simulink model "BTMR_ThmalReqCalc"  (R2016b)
settings: Solver=FixedStepDiscrete  StartTime=0.0  StopTime=10.0  FixedStep=0.1  RelTol=1e-3  EnableMultiTasking=on
undefined symbols (not defined in the file or in its folder): BMS_cntThmStbNum_C, BTMR_cntThmalReqVal_C, BTMR_flgCoolPwrCal_C, BTMR_pChrgClntPwrLv1_C, BTMR_pChrgClntPwrLv2_C, BTMR_pChrgClntPwrLv3_C, BTMR_pChrgClntPwrLv4_C, BTMR_pChrgClntPwrLv5_C, BTMR_pChrgClntPwrLv6_C, BTMR_pCoolPwrVal_C, BTMR_pHtgACPwrReq_C, BTMR_pHtgDCPwrReq_C, BTMR_pHtgDrvPwrReq_C, BTMR_pHtgsStage1_CUR, BTMR_pHtgsStage2_CUR, BTMR_pNormClntPwrLv1_C, BTMR_pNormClntPwrLv2_C, BTMR_pNormClntPwrLv3_C, BTMR_r861BrsDrvSoc_C, BTMR_r861HtgDrvSoc_C, BTMR_r891BrsDrvSoc_C, BTMR_r891HtgDrvSoc_C, BTMR_rCoolClbFlg_C, BTMR_rFlashClbFlg_C, BTMR_rHeatClbFlg_C, BTMR_t861BrsDiffLv0Temp_C, BTMR_t861BrsDiffLv1Temp_C, BTMR_t861CoolChrgAces2Temp_C, BTMR_t861CoolChrgAces3Temp_C, BTMR_t861CoolChrgAcesTemp_C, BTMR_t861CoolChrgDiffDebTemp_C, BTMR_t861CoolChrgEndDiffTemp_C, BTMR_t861CoolChrgExitLv2Temp_C, BTMR_t861CoolChrgExitLv3Temp_C, BTMR_t861CoolChrgExitTemp_C, BTMR_t861CoolChrgIntLv0Temp_C, BTMR_t861CoolChrgIntLv1Temp_C, BTMR_t861CoolChrgIntLv2Temp_C, BTMR_t861CoolChrgIntLv3Temp_C, BTMR_t861CoolChrgIntLv4Temp_C, BTMR_t861CoolChrgIntLv5Temp_C, BTMR_t861CoolDCDebTemp_C, BTMR_t861CoolNormAcesTemp_C, BTMR_t861CoolNormDiffDebTemp_C, BTMR_t861CoolNormEndDiffTemp_C, BTMR_t861CoolNormExitLv2Temp_C, BTMR_t861CoolNormExitLv3Temp_C, BTMR_t861CoolNormExitTemp_C, BTMR_t861CoolNormIntLv0Temp_C, BTMR_t861CoolNormIntLv1Temp_C, BTMR_t861CoolNormLv2Temp_C, BTMR_t861CoolNormLv3Temp_C, BTMR_t861HtgACDiffDebTemp_C, BTMR_t861HtgACEndDiffTemp_C, BTMR_t861HtgACStartHiTemp_C, BTMR_t861HtgACStartLoTemp_C, BTMR_t861HtgACStopTemp_C, BTMR_t861HtgDCDiffDebTemp_C, BTMR_t861HtgDCEndDiffTemp_C, BTMR_t861HtgDCIntLv0Temp_C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
libraries: AIWAYS_Powertrain_BMS_lib x78, simulink x9
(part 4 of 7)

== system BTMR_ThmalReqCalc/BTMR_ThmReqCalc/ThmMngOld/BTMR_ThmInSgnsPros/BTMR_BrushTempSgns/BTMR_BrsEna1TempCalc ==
  BSPR_tCellTempMin : Inport
  BSPR_tCellTempMax : Inport  Port=2
  BMSDebounceStartZero : AIWAYS_Powertrain_BMS_lib/Debounce & Delay/BMSDebounceStartZero
  Constant13 : Constant  Value=BTMR_t861CoolChrgAcesTemp_C
  Constant17 : Constant  Value=BTMR_t861HtgDCStartHiTemp_C
  Constant29 : Constant  Value=BTMR_tiTempBase_C
  Constant30 : Constant  Value=BTMR_tiTempDebs_C
  Logical Operator2 : Logic  AllPortsSameDT=off  OutDataTypeStr=boolean
  Relational Operator8 : RelationalOperator  OutDataTypeStr=boolean  RndMeth=Simplest
  Relational Operator9 : RelationalOperator  Operator=<  OutDataTypeStr=boolean  RndMeth=Simplest
  BTMR_flgBrsEna1Temp : Outport
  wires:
  Relational Operator8/1 -> Logical Operator2/1
  Relational Operator9/1 -> Logical Operator2/2
  Constant13/1 -> Relational Operator9/2
  Constant17/1 -> Relational Operator8/2
  BSPR_tCellTempMin/1 -> Relational Operator8/1
  BSPR_tCellTempMax/1 -> Relational Operator9/1
  Logical Operator2/1 -> BMSDebounceStartZero/1
  BMSDebounceStartZero/1 -> BTMR_flgBrsEna1Temp/1
  Constant29/1 -> BMSDebounceStartZero/5, BMSDebounceStartZero/3
  Constant30/1 -> BMSDebounceStartZero/4, BMSDebounceStartZero/2

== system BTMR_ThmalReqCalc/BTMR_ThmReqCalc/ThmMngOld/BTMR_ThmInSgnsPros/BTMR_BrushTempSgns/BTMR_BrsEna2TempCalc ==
  BSPR_tCellTempMin : Inport
  BSPR_tCellTempMax : Inport  Port=2
  BMSDebounceStartZero : AIWAYS_Powertrain_BMS_lib/Debounce & Delay/BMSDebounceStartZero
  Constant14 : Constant  Value=BTMR_t861HtgACStartHiTemp_C
  Constant16 : Constant  Value=BTMR_t861CoolNormAcesTemp_C
  Constant29 : Constant  Value=BTMR_tiTempBase_C
  Constant30 : Constant  Value=BTMR_tiTempDebs_C
  Logical Operator3 : Logic  AllPortsSameDT=off  OutDataTypeStr=boolean
  Relational Operator10 : RelationalOperator  OutDataTypeStr=boolean  RndMeth=Simplest
  Relational Operator11 : RelationalOperator  Operator=<  OutDataTypeStr=boolean  RndMeth=Simplest
  BTMR_flgBrsEna2Temp : Outport
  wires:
  BMSDebounceStartZero/1 -> BTMR_flgBrsEna2Temp/1
  BSPR_tCellTempMax/1 -> Relational Operator11/1
  BSPR_tCellTempMin/1 -> Relational Operator10/1
  Logical Operator3/1 -> BMSDebounceStartZero/1
  Relational Operator10/1 -> Logical Operator3/1
  Relational Operator11/1 -> Logical Operator3/2
  Constant14/1 -> Relational Operator10/2
  Constant16/1 -> Relational Operator11/2
  Constant29/1 -> BMSDebounceStartZero/5, BMSDebounceStartZero/3
  Constant30/1 -> BMSDebounceStartZero/4, BMSDebounceStartZero/2

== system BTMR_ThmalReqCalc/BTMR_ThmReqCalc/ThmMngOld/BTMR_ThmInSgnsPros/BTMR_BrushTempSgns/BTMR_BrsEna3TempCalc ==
  BSPR_tCellTempMin : Inport
  BSPR_tCellTempMax : Inport  Port=2
  BMSDebounceStartZero : AIWAYS_Powertrain_BMS_lib/Debounce & Delay/BMSDebounceStartZero
  Constant19 : Constant  Value=BTMR_t861CoolNormAcesTemp_C
  Constant20 : Constant  Value=BTMR_t861HtgDrvStartHiTemp_C
  Constant29 : Constant  Value=BTMR_tiTempBase_C
  Constant30 : Constant  Value=BTMR_tiTempDebs_C
  Logical Operator4 : Logic  AllPortsSameDT=off  OutDataTypeStr=boolean
  Relational Operator12 : RelationalOperator  Operator=>  OutDataTypeStr=boolean  RndMeth=Simplest
  Relational Operator13 : RelationalOperator  Operator=<  OutDataTypeStr=boolean  RndMeth=Simplest
  BTMR_flgBrsEna3Temp : Outport
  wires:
  BSPR_tCellTempMax/1 -> Relational Operator13/1
  BMSDebounceStartZero/1 -> BTMR_flgBrsEna3Temp/1
  Relational Operator12/1 -> Logical Operator4/1
  Constant19/1 -> Relational Operator13/2
  Relational Operator13/1 -> Logical Operator4/2
  Constant20/1 -> Relational Operator12/2
  Logical Operator4/1 -> BMSDebounceStartZero/1
  BSPR_tCellTempMin/1 -> Relational Operator12/1
  Constant29/1 -> BMSDebounceStartZero/5, BMSDebounceStartZero/3
  Constant30/1 -> BMSDebounceStartZero/4, BMSDebounceStartZero/2

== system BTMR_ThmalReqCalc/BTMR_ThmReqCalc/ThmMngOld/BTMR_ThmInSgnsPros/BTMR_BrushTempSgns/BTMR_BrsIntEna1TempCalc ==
  BSPR_tClntUsT : Inport
  BMSDebounceStartZero : AIWAYS_Powertrain_BMS_lib/Debounce & Delay/BMSDebounceStartZero
  Constant13 : Constant  Value=BTMR_t861CoolChrgAcesTemp_C
  Constant17 : Constant  Value=BTMR_t861HtgDCStartHiTemp_C
  Constant29 : Constant  Value=BTMR_tiTempBase_C
  Constant30 : Constant  Value=BTMR_tiTempDebs_C
  Logical Operator2 : Logic  AllPortsSameDT=off  OutDataTypeStr=boolean
  Relational Operator8 : RelationalOperator  OutDataTypeStr=boolean  RndMeth=Simplest
  Relational Operator9 : RelationalOperator  Operator=<  OutDataTypeStr=boolean  RndMeth=Simplest
  BTMR_flgBrsIntEna1Temp : Outport
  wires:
  BMSDebounceStartZero/1 -> BTMR_flgBrsIntEna1Temp/1
  Logical Operator2/1 -> BMSDebounceStartZero/1
  BSPR_tClntUsT/1 -> Relational Operator9/1, Relational Operator8/1
  Constant17/1 -> Relational Operator8/2
  Constant13/1 -> Relational Operator9/2
  Relational Operator9/1 -> Logical Operator2/2
  Relational Operator8/1 -> Logical Operator2/1
  Constant29/1 -> BMSDebounceStartZero/5, BMSDebounceStartZero/3
  Constant30/1 -> BMSDebounceStartZero/4, BMSDebounceStartZero/2

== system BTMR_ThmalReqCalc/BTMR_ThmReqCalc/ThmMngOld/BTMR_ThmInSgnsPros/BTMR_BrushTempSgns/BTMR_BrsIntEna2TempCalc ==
  BSPR_tClntUsT : Inport
  BMSDebounceStartZero : AIWAYS_Powertrain_BMS_lib/Debounce & Delay/BMSDebounceStartZero
  Constant14 : Constant  Value=BTMR_t861HtgACStartHiTemp_C
  Constant16 : Constant  Value=BTMR_t861CoolNormAcesTemp_C
  Constant29 : Constant  Value=BTMR_tiTempBase_C
  Constant30 : Constant  Value=BTMR_tiTempDebs_C
  Logical Operator3 : Logic  AllPortsSameDT=off  OutDataTypeStr=boolean
  Relational Operator10 : RelationalOperator  OutDataTypeStr=boolean  RndMeth=Simplest
  Relational Operator11 : RelationalOperator  Operator=<  OutDataTypeStr=boolean  RndMeth=Simplest
  BTMR_flgBrsIntEna2Temp : Outport
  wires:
  Constant16/1 -> Relational Operator11/2
  Constant14/1 -> Relational Operator10/2
  Relational Operator11/1 -> Logical Operator3/2
  Relational Operator10/1 -> Logical Operator3/1
  Logical Operator3/1 -> BMSDebounceStartZero/1
  BSPR_tClntUsT/1 -> Relational Operator11/1, Relational Operator10/1
  BMSDebounceStartZero/1 -> BTMR_flgBrsIntEna2Temp/1
  Constant29/1 -> BMSDebounceStartZero/5, BMSDebounceStartZero/3
  Constant30/1 -> BMSDebounceStartZero/4, BMSDebounceStartZero/2

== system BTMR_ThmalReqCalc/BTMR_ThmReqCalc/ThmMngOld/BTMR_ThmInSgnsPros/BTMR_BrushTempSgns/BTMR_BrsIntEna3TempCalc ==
  BSPR_tClntUsT : Inport
  BMSDebounceStartZero : AIWAYS_Powertrain_BMS_lib/Debounce & Delay/BMSDebounceStartZero
  Constant19 : Constant  Value=BTMR_t861CoolNormAcesTemp_C
  Constant20 : Constant  Value=BTMR_t861HtgDrvStartHiTemp_C
  Constant29 : Constant  Value=BTMR_tiTempBase_C
  Constant30 : Constant  Value=BTMR_tiTempDebs_C
  Logical Operator4 : Logic  AllPortsSameDT=off  OutDataTypeStr=boolean
  Relational Operator12 : RelationalOperator  Operator=>  OutDataTypeStr=boolean  RndMeth=Simplest
  Relational Operator13 : RelationalOperator  Operator=<  OutDataTypeStr=boolean  RndMeth=Simplest
  BTMR_flgBrsIntEna3Temp : Outport
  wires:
  Logical Operator4/1 -> BMSDebounceStartZero/1
  Constant20/1 -> Relational Operator12/2
  Relational Operator13/1 -> Logical Operator4/2
  Constant19/1 -> Relational Operator13/2
  Relational Operator12/1 -> Logical Operator4/1
  BMSDebounceStartZero/1 -> BTMR_flgBrsIntEna3Temp/1
  BSPR_tClntUsT/1 -> Relational Operator13/1, Relational Operator12/1
  Constant29/1 -> BMSDebounceStartZero/5, BMSDebounceStartZero/3
  Constant30/1 -> BMSDebounceStartZero/4, BMSDebounceStartZero/2

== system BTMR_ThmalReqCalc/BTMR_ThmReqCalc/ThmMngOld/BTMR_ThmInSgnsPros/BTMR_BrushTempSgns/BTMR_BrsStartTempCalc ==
  BSPR_tCellTempMin : Inport
  BSPR_tCellTempMax : Inport  Port=2
  BSPR_tClntUsT : Inport  Port=3
  Add : Sum  Inputs=+-
  Add1 : Sum  Inputs=+-
  Add2 : Sum  Inputs=+-
  BMSDebounceStartZero : AIWAYS_Powertrain_BMS_lib/Debounce & Delay/BMSDebounceStartZero
  Constant1 : Constant  Value=BTMR_tBrsCellClntDvtTemp_C
  Constant2 : Constant  Value=BTMR_t861BrsDiffLv1Temp_C
  Constant29 : Constant  Value=BTMR_tiTempBase_C
  Constant3 : Constant  Value=BTMR_tBrsMinCellTempThre_C
  Constant30 : Constant  Value=BTMR_tiTempDebs_C
  Constant4 : Constant  Value=BTMR_tBrsCellClntDvtTemp_C
  Logical Operator4 : Logic  Inputs=4  AllPortsSameDT=off  OutDataTypeStr=boolean
  Relational Operator1 : RelationalOperator  Operator=<  OutDataTypeStr=boolean  RndMeth=Simplest
  Relational Operator2 : RelationalOperator  OutDataTypeStr=boolean  RndMeth=Simplest
  Relational Operator3 : RelationalOperator  Operator=<  OutDataTypeStr=boolean  RndMeth=Simplest
  Relational Operator4 : RelationalOperator  OutDataTypeStr=boolean  RndMeth=Simplest
  BTMR_flgBrsStartTemp : Outport
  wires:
  BMSDebounceStartZero/1 -> BTMR_flgBrsStartTemp/1
  Add/1 -> Relational Operator2/1
  Constant2/1 -> Relational Operator2/2
  Relational Operator2/1 -> Logical Operator4/1
  BSPR_tCellTempMax/1 -> Add2/2, Add/1
  BSPR_tCellTempMin/1 -> Relational Operator4/1, Add/2, Add1/1
  Constant29/1 -> BMSDebounceStartZero/5, BMSDebounceStartZero/3
  Constant30/1 -> BMSDebounceStartZero/4, BMSDebounceStartZero/2
  Relational Operator1/1 -> Logical Operator4/2
  Constant1/1 -> Relational Operator1/2
  Relational Operator3/1 -> Logical Operator4/3
  Add1/1 -> Relational Operator1/1
  Constant4/1 -> Relational Operator3/2
  Add2/1 -> Relational Operator3/1
  BSPR_tClntUsT/1 -> Add2/1, Add1/2
  Logical Operator4/1 -> BMSDebounceStartZero/1
  Constant3/1 -> Relational Operator4/2
  Relational Operator4/1 -> Logical Operator4/4

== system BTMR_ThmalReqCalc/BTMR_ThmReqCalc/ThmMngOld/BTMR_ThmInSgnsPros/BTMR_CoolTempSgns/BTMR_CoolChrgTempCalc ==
  BSPR_tCellTempMax : Inport
  BSPR_tClntUsT : Inport  Port=2
  BTMR_CoolChrgInTempCalc : Subsystem
  BTMR_CoolChrgIntTempCalc : Subsystem
  Bus Creator : BusCreator  Inputs=2
  BTMR_flgCoolChrgTempSgns : Outport
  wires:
  BSPR_tClntUsT/1 -> BTMR_CoolChrgIntTempCalc/1(BSPR_tClntUsT)
  BSPR_tCellTempMax/1 -> BTMR_CoolChrgInTempCalc/1(BSPR_tCellTempMax)
  BTMR_CoolChrgInTempCalc/1(BTMR_flgCoolChrgInTempSgns) -> Bus Creator/1
  BTMR_CoolChrgIntTempCalc/1(BTMR_flgCoolChrgIntTempSgns) -> Bus Creator/2
  Bus Creator/1 -> BTMR_flgCoolChrgTempSgns/1  "BTMR_flgCoolChrgTempSgns"

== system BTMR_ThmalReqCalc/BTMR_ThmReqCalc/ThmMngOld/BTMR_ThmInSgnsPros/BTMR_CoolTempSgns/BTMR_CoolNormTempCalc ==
  BSPR_tCellTempMax : Inport
  BSPR_tClntUsT : Inport  Port=2
  BTMR_CoolNormInTempCalc : Subsystem
  BTMR_CoolNormIntTempCalc : Subsystem
  Bus Creator2 : BusCreator  Inputs=2
  BTMR_flgCoolNormTempSgns : Outport
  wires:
  Bus Creator2/1 -> BTMR_flgCoolNormTempSgns/1  "BTMR_flgCoolNormTempSgns"
  BSPR_tCellTempMax/1 -> BTMR_CoolNormInTempCalc/1(BSPR_tCellTempMax)
  BTMR_CoolNormInTempCalc/1(BTMR_flgCoolNormInTempSgns) -> Bus Creator2/1
  BSPR_tClntUsT/1 -> BTMR_CoolNormIntTempCalc/1(BSPR_tClntUsT)
  BTMR_CoolNormIntTempCalc/1(BTMR_flgCoolNormIntTempSgns) -> Bus Creator2/2

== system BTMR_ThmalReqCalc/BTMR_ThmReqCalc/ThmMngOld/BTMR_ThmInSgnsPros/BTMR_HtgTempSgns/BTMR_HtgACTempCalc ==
  BSPR_tCellTempMin : Inport
  BTMR_HtgACDnaTempCalc : Subsystem
  Bus Creator : BusCreator  Inputs=1
  BTMR_flgHtgACTempSgns : Outport
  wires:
  BTMR_HtgACDnaTempCalc/1(BTMR_flgHtgACDnaTemp) -> Bus Creator/1  "BTMR_flgHtgACDnaTemp"
  BSPR_tCellTempMin/1 -> BTMR_HtgACDnaTempCalc/1(BSPR_tCellTempMin)
  Bus Creator/1 -> BTMR_flgHtgACTempSgns/1  "BTMR_flgHtgACTempSgns"

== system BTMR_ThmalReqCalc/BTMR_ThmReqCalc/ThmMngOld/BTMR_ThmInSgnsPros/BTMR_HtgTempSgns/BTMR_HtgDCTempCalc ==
  BSPR_tCellTempMin : Inport
  BSPR_tCellTempMax : Inport  Port=2
  BSPR_tClntUsT : Inport  Port=3
  BTMR_HtgDCDnaTempCalc : Subsystem
  BTMR_HtgDCStage2EnaTempCalc : Subsystem
  BTMR_HtgDCStage2PowRedTempCalc : Subsystem
  BTMR_HtgDCStage2PowResTempCalc : Subsystem
  BTMR_HtgDCStage3EnaTempCalc : Subsystem
  BTMR_HtgDCStage3PowRedTempCalc : Subsystem
  BTMR_HtgDCStage3PowResTempCalc : Subsystem
  Bus Creator : BusCreator  Inputs=2
  Bus Creator1 : BusCreator  Inputs=5
  Bus Creator2 : BusCreator  Inputs=2
  BTMR_flgHtgDCTempSgns : Outport
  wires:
  BSPR_tClntUsT/1 -> BTMR_HtgDCStage2PowRedTempCalc/1(BSPR_tClntUsT), BTMR_HtgDCStage3PowResTempCalc/1(BSPR_tClntUsT), BTMR_HtgDCStage3PowRedTempCalc/1(BSPR_tClntUsT), BTMR_HtgDCStage2PowResTempCalc/1(BSPR_tClntUsT), BTMR_HtgDCStage2EnaTempCalc/1(BSPR_tClntUsT)
  BSPR_tCellTempMax/1 -> BTMR_HtgDCDnaTempCalc/2(BSPR_tCellTempMax), BTMR_HtgDCStage3EnaTempCalc/2(BSPR_tCellTempMax)
  BTMR_HtgDCDnaTempCalc/1(BTMR_flgHtgDCDnaTemp) -> Bus Creator/2  "BTMR_flgHtgDCDnaTemp"
  BTMR_HtgDCStage3EnaTempCalc/1(BTMR_flgHtgDCStage3EnaTemp) -> Bus Creator/1  "BTMR_flgHtgDCStage3EnaTemp"
  BTMR_HtgDCStage2EnaTempCalc/1(BTMR_flgHtgDCStage2EnaTemp) -> Bus Creator1/1  "BTMR_flgHtgDCStage2EnaTemp"
  BSPR_tCellTempMin/1 -> BTMR_HtgDCDnaTempCalc/1(BSPR_tCellTempMin), BTMR_HtgDCStage3EnaTempCalc/1(BSPR_tCellTempMin)
  BTMR_HtgDCStage2PowRedTempCalc/1(BTMR_flgHtgDCStage2PowRedTemp) -> Bus Creator1/2  "BTMR_HtgDCStage2PowRedTemp"
  BTMR_HtgDCStage2PowResTempCalc/1(BTMR_flgHtgDCStage2PowResTemp) -> Bus Creator1/3  "BTMR_HtgDCStage2PowResTemp"
  BTMR_HtgDCStage3PowRedTempCalc/1(BTMR_flgHtgDCStage3PowRedTemp) -> Bus Creator1/4  "BTMR_HtgDCStage3PowRedTemp"
  BTMR_HtgDCStage3PowResTempCalc/1(BTMR_flgHtgDCStage3PowResTemp) -> Bus Creator1/5  "BTMR_HtgDCStage3PowResTemp"
  Bus Creator/1 -> Bus Creator2/1  "BTMR_flgHtgDCInTempSgns"
  Bus Creator1/1 -> Bus Creator2/2  "BTMR_flgHtgDCIntTempSgns"
  Bus Creator2/1 -> BTMR_flgHtgDCTempSgns/1  "BTMR_flgHtgDCTempSgns"

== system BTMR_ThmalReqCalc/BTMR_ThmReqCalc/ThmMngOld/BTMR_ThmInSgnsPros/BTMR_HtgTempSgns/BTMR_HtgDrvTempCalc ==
  BSPR_tCellTempMin : Inport
  BTMR_HtgDrvDnaTempCalc : Subsystem
  Bus Creator : BusCreator  Inputs=1
  BTMR_flgHtgDrvTempSgns : Outport
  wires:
  BTMR_HtgDrvDnaTempCalc/1(BTMR_flgHtgDrvDnaTemp) -> Bus Creator/1  "BTMR_flgHtgDrvDnaTemp"
  BSPR_tCellTempMin/1 -> BTMR_HtgDrvDnaTempCalc/1(BSPR_tCellTempMin)
  Bus Creator/1 -> BTMR_flgHtgDrvTempSgns/1  "BTMR_flgHtgDrvTempSgns"

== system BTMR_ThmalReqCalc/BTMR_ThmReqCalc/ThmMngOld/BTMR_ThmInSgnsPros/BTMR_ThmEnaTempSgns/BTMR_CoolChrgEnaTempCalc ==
  BSPR_tCellTempMin : Inport
  BSPR_tCellTempMax : Inport  Port=2
  Add : Sum
  Add1 : Sum  Inputs=+-
  Add2 : Sum  Inputs=+-
  BMSDebounceStartZero : AIWAYS_Powertrain_BMS_lib/Debounce & Delay/BMSDebounceStartZero
  Constant1 : Constant  Value=BTMR_t861HtgDCStopTemp_C
  Constant2 : Constant  Value=BTMR_t861CoolDCDebTemp_C
  Constant27 : Constant  Value=BTMR_t861CoolChrgAcesTemp_C
  Constant29 : Constant  Value=BTMR_tiTempBase_C
  Constant3 : Constant  Value=BTMR_t861CoolChrgDiffDebTemp_C
  Constant30 : Constant  Value=BTMR_tiTempDebs_C
  Constant4 : Constant  Value=BTMR_t861CoolChrgEndDiffTemp_C
  Logical Operator : Logic  Inputs=3  AllPortsSameDT=off  OutDataTypeStr=boolean
  Relational Operator1 : RelationalOperator  OutDataTypeStr=boolean  RndMeth=Simplest
  Relational Operator19 : RelationalOperator  OutDataTypeStr=boolean  RndMeth=Simplest
  Relational Operator2 : RelationalOperator  Operator=<  OutDataTypeStr=boolean  RndMeth=Simplest
  BTMR_flgCoolChrgEnaTemp : Outport
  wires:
  Logical Operator/1 -> BMSDebounceStartZero/1
  BSPR_tCellTempMax/1 -> Relational Operator19/1, Add1/1
  Constant27/1 -> Relational Operator19/2
  BMSDebounceStartZero/1 -> BTMR_flgCoolChrgEnaTemp/1
  Constant29/1 -> BMSDebounceStartZero/5, BMSDebounceStartZero/3
  Constant30/1 -> BMSDebounceStartZero/4, BMSDebounceStartZero/2
  BSPR_tCellTempMin/1 -> Relational Operator1/1, Add1/2
  Add/1 -> Relational Operator1/2
  Constant2/1 -> Add/2
  Constant1/1 -> Add/1
  Relational Operator19/1 -> Logical Operator/1
  Relational Operator1/1 -> Logical Operator/3
  Constant4/1 -> Add2/1
  Add2/1 -> Relational Operator2/2
  Constant3/1 -> Add2/2
  Add1/1 -> Relational Operator2/1
  Relational Operator2/1 -> Logical Operator/2

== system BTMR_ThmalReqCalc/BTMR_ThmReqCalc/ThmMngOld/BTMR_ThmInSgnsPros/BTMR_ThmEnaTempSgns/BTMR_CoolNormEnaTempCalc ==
  BSPR_tCellTempMin : Inport
  BSPR_tCellTempMax : Inport  Port=2
  Add1 : Sum  Inputs=+-
  Add2 : Sum  Inputs=+-
  BMSDebounceStartZero : AIWAYS_Powertrain_BMS_lib/Debounce & Delay/BMSDebounceStartZero
  Constant28 : Constant  Value=BTMR_t861CoolNormAcesTemp_C
  Constant29 : Constant  Value=BTMR_tiTempBase_C
  Constant3 : Constant  Value=BTMR_t861CoolNormDiffDebTemp_C
  Constant30 : Constant  Value=BTMR_tiTempDebs_C
  Constant4 : Constant  Value=BTMR_t861CoolNormEndDiffTemp_C
  Logical Operator : Logic  AllPortsSameDT=off  OutDataTypeStr=boolean
  Relational Operator2 : RelationalOperator  Operator=<  OutDataTypeStr=boolean  RndMeth=Simplest
  Relational Operator20 : RelationalOperator  OutDataTypeStr=boolean  RndMeth=Simplest
  BTMR_flgCoolNormEnaTemp : Outport
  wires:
  BMSDebounceStartZero/1 -> BTMR_flgCoolNormEnaTemp/1  "BTMR_flgCoolNormEnaTemp"
  Constant28/1 -> Relational Operator20/2
  BSPR_tCellTempMax/1 -> Add1/1, Relational Operator20/1
  Constant29/1 -> BMSDebounceStartZero/5, BMSDebounceStartZero/3
  Constant30/1 -> BMSDebounceStartZero/4, BMSDebounceStartZero/2
  Add2/1 -> Relational Operator2/2
  BSPR_tCellTempMin/1 -> Add1/2
  Constant3/1 -> Add2/2
  Add1/1 -> Relational Operator2/1
  Constant4/1 -> Add2/1
  Relational Operator20/1 -> Logical Operator/1
  Relational Operator2/1 -> Logical Operator/2  "BTMR_flgTempDiff"
  Logical Operator/1 -> BMSDebounceStartZero/1

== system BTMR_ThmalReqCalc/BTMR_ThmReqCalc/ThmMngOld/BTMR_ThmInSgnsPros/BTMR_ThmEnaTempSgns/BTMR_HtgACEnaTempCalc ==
  BSPR_tCellTempMin : Inport
  BSPR_tCellTempMax : Inport  Port=2
  BMSDebounceStartZero : AIWAYS_Powertrain_BMS_lib/Debounce & Delay/BMSDebounceStartZero
  Constant1 : Constant  Value=BTMR_t861HtgACDiffDebTemp_C
  Constant2 : Constant  Value=BTMR_t861HtgACEndDiffTemp_C
  Constant23 : Constant  Value=BTMR_t861HtgACStartLoTemp_C
  Constant24 : Constant  Value=BTMR_t861HtgACStartHiTemp_C
  Constant29 : Constant  Value=BTMR_tiTempBase_C
  Constant30 : Constant  Value=BTMR_tiTempDebs_C
  Logical Operator6 : Logic  Inputs=3  AllPortsSameDT=off  OutDataTypeStr=boolean
  Relational Operator1 : RelationalOperator  Operator=<  OutDataTypeStr=boolean  RndMeth=Simplest
  Relational Operator14 : RelationalOperator  OutDataTypeStr=boolean  RndMeth=Simplest
  Relational Operator15 : RelationalOperator  Operator=<  OutDataTypeStr=boolean  RndMeth=Simplest
  Sum1 : Sum  Inputs=+-  OutDataTypeStr=Inherit: Inherit via back propagation  RndMeth=Zero
  Sum2 : Sum  Inputs=+-  OutDataTypeStr=Inherit: Inherit via back propagation  RndMeth=Zero
  BTMR_flgHtgACEnaTemp : Outport
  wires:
  BMSDebounceStartZero/1 -> BTMR_flgHtgACEnaTemp/1
  Relational Operator14/1 -> Logical Operator6/2
  Constant24/1 -> Relational Operator15/2
  Constant23/1 -> Relational Operator14/2
  Relational Operator15/1 -> Logical Operator6/3
  Logical Operator6/1 -> BMSDebounceStartZero/1
  Constant29/1 -> BMSDebounceStartZero/5, BMSDebounceStartZero/3
  Constant30/1 -> BMSDebounceStartZero/4, BMSDebounceStartZero/2
  Sum2/1 -> Relational Operator1/2
  Constant1/1 -> Sum2/2
  BSPR_tCellTempMax/1 -> Sum1/1
  Sum1/1 -> Relational Operator1/1
  BSPR_tCellTempMin/1 -> Sum1/2, Relational Operator15/1, Relational Operator14/1
  Relational Operator1/1 -> Logical Operator6/1
  Constant2/1 -> Sum2/1

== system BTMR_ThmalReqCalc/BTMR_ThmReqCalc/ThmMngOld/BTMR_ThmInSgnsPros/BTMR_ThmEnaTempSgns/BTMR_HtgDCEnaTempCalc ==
  BSPR_tCellTempMin : Inport
  BSPR_tCellTempMax : Inport  Port=2
  BMSDebounceStartZero : AIWAYS_Powertrain_BMS_lib/Debounce & Delay/BMSDebounceStartZero
  Constant1 : Constant  Value=BTMR_t861HtgDCDiffDebTemp_C
  Constant2 : Constant  Value=BTMR_t861HtgDCEndDiffTemp_C
  Constant23 : Constant  Value=BTMR_t861HtgDCStopTemp2_C
  Constant25 : Constant  Value=BTMR_t861HtgDCStartHiTemp_C
  Constant26 : Constant  Value=BTMR_t861HtgDCStartLoTemp_C
  Constant29 : Constant  Value=BTMR_tiTempBase_C
  Constant30 : Constant  Value=BTMR_tiTempDebs_C
  Constant5 : Constant  Value=BTMR_tHtgDCMaxTempDeb_C
  Logical Operator6 : Logic  Inputs=4  AllPortsSameDT=off  OutDataTypeStr=boolean
  Relational Operator1 : RelationalOperator  Operator=<  OutDataTypeStr=boolean  RndMeth=Simplest
  Relational Operator16 : RelationalOperator  Operator=>  OutDataTypeStr=boolean  RndMeth=Simplest
  Relational Operator17 : RelationalOperator  Operator=<  OutDataTypeStr=boolean  RndMeth=Simplest
  Relational Operator2 : RelationalOperator  Operator=<  OutDataTypeStr=boolean  RndMeth=Simplest
  Sum1 : Sum  Inputs=+-  OutDataTypeStr=Inherit: Inherit via back propagation  RndMeth=Zero
  Sum2 : Sum  Inputs=+-  OutDataTypeStr=Inherit: Inherit via back propagation  RndMeth=Zero
  Sum3 : Sum  Inputs=+-  OutDataTypeStr=Inherit: Inherit via back propagation  RndMeth=Zero
  BTMR_flgHtgDCEnaTemp : Outport
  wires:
  BMSDebounceStartZero/1 -> BTMR_flgHtgDCEnaTemp/1
  BSPR_tCellTempMin/1 -> Sum1/2, Relational Operator17/1, Relational Operator16/1
  Constant25/1 -> Relational Operator17/2
  Relational Operator17/1 -> Logical Operator6/4
  Constant26/1 -> Relational Operator16/2
  Relational Operator16/1 -> Logical Operator6/3
  Logical Operator6/1 -> BMSDebounceStartZero/1
  Constant30/1 -> BMSDebounceStartZero/4, BMSDebounceStartZero/2
  Constant29/1 -> BMSDebounceStartZero/5, BMSDebounceStartZero/3
  Sum1/1 -> Relational Operator1/1
  Constant1/1 -> Sum2/2
  Constant2/1 -> Sum2/1
  Sum2/1 -> Relational Operator1/2
  Relational Operator1/1 -> Logical Operator6/2
  Sum3/1 -> Relational Operator2/2
  Constant5/1 -> Sum3/2
  Constant23/1 -> Sum3/1
  BSPR_tCellTempMax/1 -> Relational Operator2/1, Sum1/1
  Relational Operator2/1 -> Logical Operator6/1

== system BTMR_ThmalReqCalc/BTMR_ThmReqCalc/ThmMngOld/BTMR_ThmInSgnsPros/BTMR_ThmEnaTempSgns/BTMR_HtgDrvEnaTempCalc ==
  BSPR_tCellTempMin : Inport
  BSPR_tCellTempMax : Inport  Port=2
  BMSDebounceStartZero : AIWAYS_Powertrain_BMS_lib/Debounce & Delay/BMSDebounceStartZero
  Constant1 : Constant  Value=BTMR_t861HtgDrvDiffDebTemp_C
  Constant2 : Constant  Value=BTMR_t861HtgDrvEndDiffTemp_C
  Constant21 : Constant  Value=BTMR_t861HtgDrvStartLoTemp_C
  Constant22 : Constant  Value=BTMR_t861HtgDrvStartHiTemp_C
  Constant29 : Constant  Value=BTMR_tiTempBase_C
  Constant30 : Constant  Value=BTMR_tiTempDebs_C
  Logical Operator6 : Logic  Inputs=3  AllPortsSameDT=off  OutDataTypeStr=boolean
  Relational Operator1 : RelationalOperator  OutDataTypeStr=boolean  RndMeth=Simplest
  Relational Operator18 : RelationalOperator  Operator=<=  OutDataTypeStr=boolean  RndMeth=Simplest
  Relational Operator2 : RelationalOperator  Operator=<  OutDataTypeStr=boolean  RndMeth=Simplest
  Sum1 : Sum  Inputs=+-  OutDataTypeStr=Inherit: Inherit via back propagation  RndMeth=Zero
  Sum2 : Sum  Inputs=+-  OutDataTypeStr=Inherit: Inherit via back propagation  RndMeth=Zero
  BTMR_flgHtgDrvEnaTemp : Outport
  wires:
  Constant22/1 -> Relational Operator18/2
  BMSDebounceStartZero/1 -> BTMR_flgHtgDrvEnaTemp/1
  Logical Operator6/1 -> BMSDebounceStartZero/1
  Constant21/1 -> Relational Operator1/2
  Relational Operator18/1 -> Logical Operator6/2
  Relational Operator1/1 -> Logical Operator6/3
  Constant29/1 -> BMSDebounceStartZero/5, BMSDebounceStartZero/3
  Constant30/1 -> BMSDebounceStartZero/4, BMSDebounceStartZero/2
  BSPR_tCellTempMax/1 -> Sum1/1
  Sum1/1 -> Relational Operator2/1
  Constant2/1 -> Sum2/1
  Sum2/1 -> Relational Operator2/2
  Constant1/1 -> Sum2/2
  BSPR_tCellTempMin/1 -> Relational Operator18/1, Sum1/2, Relational Operator1/1
  Relational Operator2/1 -> Logical Operator6/1

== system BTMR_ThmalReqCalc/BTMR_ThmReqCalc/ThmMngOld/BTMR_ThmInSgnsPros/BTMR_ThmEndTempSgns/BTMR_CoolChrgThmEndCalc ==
  BTMR_flgBMSSgns : Inport
  BSPR_tCellTempMax : Inport  Port=2
  BSPR_tCellTempMin : Inport  Port=3
  Add : Sum  Inputs=+-
  BMSDebounceStartZero : AIWAYS_Powertrain_BMS_lib/Debounce & Delay/BMSDebounceStartZero
  Bus Selector : BusSelector  OutputSignals=BTMR_flgBMSDChrg
  Constant14 : Constant  Value=BTMR_t861CoolChrgEndDiffTemp_C
  Constant29 : Constant  Value=BTMR_tiTempBase_C
  Constant30 : Constant  Value=BTMR_tiTempDebs_C
  Logical Operator1 : Logic  AllPortsSameDT=off  OutDataTypeStr=boolean
  Relational Operator3 : RelationalOperator  OutDataTypeStr=boolean  RndMeth=Simplest
  BTMR_CoolChrgThmEnd : Outport
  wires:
  BMSDebounceStartZero/1 -> Logical Operator1/2
  BSPR_tCellTempMin/1 -> Add/2
  Add/1 -> Relational Operator3/1
  Constant14/1 -> Relational Operator3/2
  BSPR_tCellTempMax/1 -> Add/1
  Relational Operator3/1 -> BMSDebounceStartZero/1
  BTMR_flgBMSSgns/1 -> Bus Selector/1
  Bus Selector/1 -> Logical Operator1/1  "<BTMR_flgBMSDChrg>"
  Logical Operator1/1 -> BTMR_CoolChrgThmEnd/1
  Constant29/1 -> BMSDebounceStartZero/5, BMSDebounceStartZero/3
  Constant30/1 -> BMSDebounceStartZero/4, BMSDebounceStartZero/2

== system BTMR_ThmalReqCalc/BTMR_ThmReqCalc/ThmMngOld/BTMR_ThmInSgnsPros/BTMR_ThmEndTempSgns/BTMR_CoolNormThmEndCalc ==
  BTMR_flgBMSSgns : Inport
  BSPR_tCellTempMax : Inport  Port=2
  BSPR_tCellTempMin : Inport  Port=3
  Add : Sum  Inputs=+-
  BMSDebounceStartZero : AIWAYS_Powertrain_BMS_lib/Debounce & Delay/BMSDebounceStartZero
  Bus Selector : BusSelector  OutputSignals=BTMR_flgBMSAChrg,BTMR_flgBMSDrv
  Constant14 : Constant  Value=BTMR_t861CoolNormEndDiffTemp_C
  Constant29 : Constant  Value=BTMR_tiTempBase_C
  Constant30 : Constant  Value=BTMR_tiTempDebs_C
  Logical Operator1 : Logic  AllPortsSameDT=off  OutDataTypeStr=boolean
  Logical Operator2 : Logic  Operator=OR  AllPortsSameDT=off  OutDataTypeStr=boolean
  Relational Operator3 : RelationalOperator  OutDataTypeStr=boolean  RndMeth=Simplest
  BTMR_CoolNormThmEnd : Outport
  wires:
  BTMR_flgBMSSgns/1 -> Bus Selector/1
  Relational Operator3/1 -> BMSDebounceStartZero/1
  BSPR_tCellTempMax/1 -> Add/1
  Constant14/1 -> Relational Operator3/2
  Add/1 -> Relational Operator3/1
  BSPR_tCellTempMin/1 -> Add/2
  BMSDebounceStartZero/1 -> Logical Operator1/2
  Bus Selector/1 -> Logical Operator2/1  "<BTMR_flgBMSAChrg>"
  Bus Selector/2 -> Logical Operator2/2  "<BTMR_flgBMSDrv>"
  Logical Operator2/1 -> Logical Operator1/1
  Logical Operator1/1 -> BTMR_CoolNormThmEnd/1
  Constant29/1 -> BMSDebounceStartZero/5, BMSDebounceStartZero/3
  Constant30/1 -> BMSDebounceStartZero/4, BMSDebounceStartZero/2

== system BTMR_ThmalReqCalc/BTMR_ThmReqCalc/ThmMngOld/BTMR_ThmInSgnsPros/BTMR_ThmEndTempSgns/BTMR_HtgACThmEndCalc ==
  BTMR_flgBMSSgns : Inport
  BSPR_tCellTempMax : Inport  Port=2
  BSPR_tCellTempMin : Inport  Port=3
  BCMR_bAcChrgHeatFbd : Inport  Port=4
  Add : Sum  Inputs=+-
  BMSDebounceStartZero : AIWAYS_Powertrain_BMS_lib/Debounce & Delay/BMSDebounceStartZero
  Bus Selector : BusSelector  OutputSignals=BTMR_flgBMSAChrg
  Constant14 : Constant  Value=BTMR_t861HtgACEndDiffTemp_C
  Constant29 : Constant  Value=BTMR_tiTempBase_C
  Constant30 : Constant  Value=BTMR_tiTempDebs_C
  Logical Operator1 : Logic  AllPortsSameDT=off  OutDataTypeStr=boolean
  Logical Operator3 : Logic  Operator=OR  AllPortsSameDT=off  OutDataTypeStr=boolean
  Relational Operator3 : RelationalOperator  OutDataTypeStr=boolean  RndMeth=Simplest
  BTMR_HtgACThmEnd : Outport
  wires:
  BMSDebounceStartZero/1 -> Logical Operator3/1
  BSPR_tCellTempMin/1 -> Add/2
  Add/1 -> Relational Operator3/1
  Constant14/1 -> Relational Operator3/2
  BSPR_tCellTempMax/1 -> Add/1
  Relational Operator3/1 -> BMSDebounceStartZero/1
  BTMR_flgBMSSgns/1 -> Bus Selector/1
  Bus Selector/1 -> Logical Operator1/1  "<BTMR_flgBMSAChrg>"
  BCMR_bAcChrgHeatFbd/1 -> Logical Operator3/2
  Logical Operator3/1 -> Logical Operator1/2
  Logical Operator1/1 -> BTMR_HtgACThmEnd/1
  Constant29/1 -> BMSDebounceStartZero/3, BMSDebounceStartZero/5
  Constant30/1 -> BMSDebounceStartZero/2, BMSDebounceStartZero/4

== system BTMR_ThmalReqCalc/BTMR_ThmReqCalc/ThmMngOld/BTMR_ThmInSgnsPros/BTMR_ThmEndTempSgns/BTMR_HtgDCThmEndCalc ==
  BTMR_flgBMSSgns : Inport
  BSPR_tCellTempMax : Inport  Port=2
  BSPR_tCellTempMin : Inport  Port=3
  Add : Sum  Inputs=+-
  BMSDebounceStartZero : AIWAYS_Powertrain_BMS_lib/Debounce & Delay/BMSDebounceStartZero
  Bus Selector : BusSelector  OutputSignals=BTMR_flgBMSDChrg
  Constant14 : Constant  Value=BTMR_t861HtgDCEndDiffTemp_C
  Constant29 : Constant  Value=BTMR_tiTempBase_C
  Constant30 : Constant  Value=BTMR_tiTempDebs_C
  Logical Operator1 : Logic  AllPortsSameDT=off  OutDataTypeStr=boolean
  Relational Operator3 : RelationalOperator  OutDataTypeStr=boolean  RndMeth=Simplest
  BTMR_HtgDCThmEnd : Outport
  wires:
  Bus Selector/1 -> Logical Operator1/1  "<BTMR_flgBMSDChrg>"
  BTMR_flgBMSSgns/1 -> Bus Selector/1
  Relational Operator3/1 -> BMSDebounceStartZero/1
  BSPR_tCellTempMax/1 -> Add/1
  Constant14/1 -> Relational Operator3/2
  Add/1 -> Relational Operator3/1
  BSPR_tCellTempMin/1 -> Add/2
  Logical Operator1/1 -> BTMR_HtgDCThmEnd/1
  BMSDebounceStartZero/1 -> Logical Operator1/2
  Constant29/1 -> BMSDebounceStartZero/5, BMSDebounceStartZero/3
  Constant30/1 -> BMSDebounceStartZero/4, BMSDebounceStartZero/2

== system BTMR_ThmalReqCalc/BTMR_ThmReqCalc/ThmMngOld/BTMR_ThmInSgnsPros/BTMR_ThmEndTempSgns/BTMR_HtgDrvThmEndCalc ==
  BTMR_flgBMSSgns : Inport
  BSPR_tCellTempMax : Inport  Port=2
  BSPR_tCellTempMin : Inport  Port=3
  Add : Sum  Inputs=+-
  BMSDebounceStartZero : AIWAYS_Powertrain_BMS_lib/Debounce & Delay/BMSDebounceStartZero
  Bus Selector : BusSelector  OutputSignals=BTMR_flgBMSDrv
  Constant14 : Constant  Value=BTMR_t861HtgDrvEndDiffTemp_C
  Constant29 : Constant  Value=BTMR_tiTempBase_C
  Constant30 : Constant  Value=BTMR_tiTempDebs_C
  Logical Operator1 : Logic  AllPortsSameDT=off  OutDataTypeStr=boolean
  Relational Operator3 : RelationalOperator  OutDataTypeStr=boolean  RndMeth=Simplest
  BTMR_HtgDrvThmEnd : Outport
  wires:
  BMSDebounceStartZero/1 -> Logical Operator1/2
  Logical Operator1/1 -> BTMR_HtgDrvThmEnd/1
  BSPR_tCellTempMin/1 -> Add/2
  Add/1 -> Relational Operator3/1
  Constant14/1 -> Relational Operator3/2
  BSPR_tCellTempMax/1 -> Add/1
  Relational Operator3/1 -> BMSDebounceStartZero/1
  BTMR_flgBMSSgns/1 -> Bus Selector/1
  Bus Selector/1 -> Logical Operator1/1  "<BTMR_flgBMSDrv>"
  Constant29/1 -> BMSDebounceStartZero/5, BMSDebounceStartZero/3
  Constant30/1 -> BMSDebounceStartZero/4, BMSDebounceStartZero/2

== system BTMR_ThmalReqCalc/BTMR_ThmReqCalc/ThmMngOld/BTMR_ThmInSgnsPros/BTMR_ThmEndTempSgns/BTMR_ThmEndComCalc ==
  BMCR_stBmsModeCtrl : Inport
  DSMR_stFaultRank : Inport  Port=2
  COMR_bLeadAcidChgHvOn : Inport  Port=3
  Data Type Conversion2 : DataTypeConversion  OutDataTypeStr=uint8
  Detect Change : simulink/Logic and Bit Operations/Detect Change  vinit=0  OutDataTypeStr=boolean
  Logical Operator10 : Logic  Operator=OR  Inputs=3  AllPortsSameDT=off  OutDataTypeStr=boolean
  Relational Operator2 : RelationalOperator  OutDataTypeStr=boolean  RndMeth=Simplest
  stBms_DChrg2 : Constant  Value=enmBmsFaultLvl.FaultLv3  OutDataTypeStr=Enum: enmBmsFaultLvl
  BTMR_ThmEndCom : Outport
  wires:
  DSMR_stFaultRank/1 -> Relational Operator2/1
  Relational Operator2/1 -> Logical Operator10/2
  Data Type Conversion2/1 -> Relational Operator2/2
  Logical Operator10/1 -> BTMR_ThmEndCom/1
  COMR_bLeadAcidChgHvOn/1 -> Logical Operator10/3
  stBms_DChrg2/1 -> Data Type Conversion2/1
  Detect Change/1 -> Logical Operator10/1
  BMCR_stBmsModeCtrl/1 -> Detect Change/1

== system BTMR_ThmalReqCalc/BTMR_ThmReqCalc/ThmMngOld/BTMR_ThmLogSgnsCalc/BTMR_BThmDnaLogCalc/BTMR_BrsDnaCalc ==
  BTMR_flgBrsLogSgns : Inport
  Bus Selector : BusSelector  OutputSignals=BTMR_flgBrsInTempSgns
  Bus Selector2 : BusSelector  OutputSignals=BTMR_flgBrsDnaTemp
  BTMR_flgBrsDna : Outport
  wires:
  Bus Selector2/1 -> BTMR_flgBrsDna/1  "<BTMR_flgBrsDnaTemp>"
  BTMR_flgBrsLogSgns/1 -> Bus Selector/1
  Bus Selector/1 -> Bus Selector2/1  "<BTMR_flgBrsInTempSgns>"

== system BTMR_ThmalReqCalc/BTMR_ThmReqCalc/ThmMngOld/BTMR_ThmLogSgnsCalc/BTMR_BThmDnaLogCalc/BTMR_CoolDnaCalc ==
  BTMR_flgCoolLogSgns : Inport
  Bus Selector : BusSelector  OutputSignals=BTMR_flgCoolNormTempSgns
  Bus Selector1 : BusSelector  OutputSignals=BTMR_flgCoolNormInTempSgns
  Bus Selector2 : BusSelector  OutputSignals=BTMR_flgCoolChrgTempSgns
  Bus Selector3 : BusSelector  OutputSignals=BTMR_flgCoolChrgInTempSgns
  Bus Selector4 : BusSelector  OutputSignals=BTMR_flgCoolNormDnaTemp
  Bus Selector5 : BusSelector  OutputSignals=BTMR_flgCoolChrgDnaTemp
  BTMR_flgCoolNormDna : Outport
  BTMR_flgCoolChrgDna : Outport  Port=2
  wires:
  Bus Selector3/1 -> Bus Selector5/1  "<BTMR_flgCoolChrgInTempSgns>"
  Bus Selector2/1 -> Bus Selector3/1  "<BTMR_flgCoolChrgTempSgns>"
  Bus Selector/1 -> Bus Selector1/1  "<BTMR_flgCoolNormTempSgns>"
  BTMR_flgCoolLogSgns/1 -> Bus Selector/1, Bus Selector2/1
  Bus Selector1/1 -> Bus Selector4/1  "<BTMR_flgCoolNormInTempSgns>"
  Bus Selector4/1 -> BTMR_flgCoolNormDna/1  "<BTMR_flgCoolNormDnaTemp>"
  Bus Selector5/1 -> BTMR_flgCoolChrgDna/1  "<BTMR_flgCoolChrgDnaTemp>"

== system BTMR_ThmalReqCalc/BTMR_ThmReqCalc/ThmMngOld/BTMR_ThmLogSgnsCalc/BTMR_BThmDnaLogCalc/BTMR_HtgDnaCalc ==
  BTMR_flgHtgLogSgns : Inport
  BTMR_flgSOCSgns : Inport  Port=2
  Bus Selector : BusSelector  OutputSignals=BTMR_flgHtgDCTempSgns
  Bus Selector1 : BusSelector  OutputSignals=BTMR_flgHtgDCInTempSgns.BTMR_flgHtgDCDnaTemp
  Bus Selector2 : BusSelector  OutputSignals=BTMR_flgHtgACTempSgns
  Bus Selector3 : BusSelector  OutputSignals=BTMR_flgHtgACDnaTemp
  Bus Selector4 : BusSelector  OutputSignals=BTMR_flgHtgDrvTempSgns
  Bus Selector5 : BusSelector  OutputSignals=BTMR_flgHtgDrvDnaTemp
  Bus Selector6 : BusSelector  OutputSignals=BTMR_flgHtgDrvSOC
  Logical Operator1 : Logic  Operator=NOT  AllPortsSameDT=off  OutDataTypeStr=boolean
  Logical Operator3 : Logic  Operator=OR  AllPortsSameDT=off  OutDataTypeStr=boolean
  BTMR_flgHtgDCDna : Outport
  BTMR_flgHtgACDna : Outport  Port=2
  BTMR_flgHtgDrvDna : Outport  Port=3
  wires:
  Bus Selector1/1 -> BTMR_flgHtgDCDna/1  "<BTMR_flgHtgDCDnaTemp>"
  Bus Selector4/1 -> Bus Selector5/1  "<BTMR_flgHtgDrvTempSgns>"
  BTMR_flgHtgLogSgns/1 -> Bus Selector2/1, Bus Selector4/1, Bus Selector/1
  Bus Selector5/1 -> Logical Operator3/1  "<BTMR_flgHtgDrvDnaTemp>"
  Bus Selector/1 -> Bus Selector1/1  "<BTMR_flgHtgDCTempSgns>"
  Bus Selector2/1 -> Bus Selector3/1  "<BTMR_flgHtgACTempSgns>"
  Bus Selector3/1 -> BTMR_flgHtgACDna/1  "<BTMR_flgHtgACDnaTemp>"
  BTMR_flgSOCSgns/1 -> Bus Selector6/1
  Bus Selector6/1 -> Logical Operator1/1  "<BTMR_flgHtgDrvSOC>"
  Logical Operator3/1 -> BTMR_flgHtgDrvDna/1
  Logical Operator1/1 -> Logical Operator3/2

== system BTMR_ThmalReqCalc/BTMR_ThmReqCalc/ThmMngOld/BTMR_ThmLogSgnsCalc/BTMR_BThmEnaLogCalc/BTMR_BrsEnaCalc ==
  BTMR_flgBrsLogSgns : Inport
  Bus Selector : BusSelector  OutputSignals=BTMR_flgBrsEnaLogSgns
  Bus Selector1 : BusSelector  OutputSignals=BTMR_flgBrsEna
  BTMR_flgBrsEna : Outport
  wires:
  BTMR_flgBrsLogSgns/1 -> Bus Selector/1
  Bus Selector/1 -> Bus Selector1/1  "<BTMR_flgBrsEnaLogSgns>"
  Bus Selector1/1 -> BTMR_flgBrsEna/1  "<BTMR_flgBrsEna>"

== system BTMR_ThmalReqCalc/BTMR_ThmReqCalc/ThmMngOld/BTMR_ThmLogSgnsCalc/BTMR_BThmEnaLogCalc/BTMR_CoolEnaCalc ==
  BTMR_flgCoolLogSgns : Inport
  Bus Selector : BusSelector  OutputSignals=BTMR_flgCoolNormLogSgns
  Bus Selector1 : BusSelector  OutputSignals=BTMR_flgCoolNormEna
  Bus Selector2 : BusSelector  OutputSignals=BTMR_flgCoolChrgLogSgns
  Bus Selector3 : BusSelector  OutputSignals=BTMR_flgCoolChrgEna
  BTMR_flgCoolNormEna : Outport
  BTMR_flgCoolChrgEna : Outport  Port=2
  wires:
  Bus Selector1/1 -> BTMR_flgCoolNormEna/1  "<BTMR_flgCoolNormEna>"
  BTMR_flgCoolLogSgns/1 -> Bus Selector2/1, Bus Selector/1
  Bus Selector/1 -> Bus Selector1/1  "<BTMR_flgCoolNormLogSgns>"
  Bus Selector2/1 -> Bus Selector3/1  "<BTMR_flgCoolChrgLogSgns>"
  Bus Selector3/1 -> BTMR_flgCoolChrgEna/1  "<BTMR_flgCoolChrgEna>"

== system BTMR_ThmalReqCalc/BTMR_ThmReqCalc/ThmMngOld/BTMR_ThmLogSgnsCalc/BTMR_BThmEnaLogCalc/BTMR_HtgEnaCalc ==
  BTMR_flgHtgLogSgns : Inport
  BTMR_flgSOCSgns : Inport  Port=2
  Bus Selector : BusSelector  OutputSignals=BTMR_flgHtgDCLogSgns
  Bus Selector1 : BusSelector  OutputSignals=BTMR_flgHtgDCEna
  Bus Selector2 : BusSelector  OutputSignals=BTMR_flgHtgACLogSgns
  Bus Selector3 : BusSelector  OutputSignals=BTMR_flgHtgACEna
  Bus Selector4 : BusSelector  OutputSignals=BTMR_flgHtgDrvLogSgns
  Bus Selector5 : BusSelector  OutputSignals=BTMR_flgHtgDrvEna
  Bus Selector6 : BusSelector  OutputSignals=BTMR_flgHtgDrvSOC
  Logical Operator : Logic  AllPortsSameDT=off  OutDataTypeStr=boolean
  BTMR_flgHtgDCEna : Outport
  BTMR_flgHtgACEna : Outport  Port=2
  BTMR_flgHtgDrvEna : Outport  Port=3
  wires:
  Bus Selector3/1 -> BTMR_flgHtgACEna/1  "<BTMR_flgHtgACEna>"
  Bus Selector2/1 -> Bus Selector3/1  "<BTMR_flgHtgACLogSgns>"
  Bus Selector/1 -> Bus Selector1/1  "<BTMR_flgHtgDCLogSgns>"
  Bus Selector5/1 -> Logical Operator/1  "<BTMR_flgHtgDrvEna>"
  BTMR_flgHtgLogSgns/1 -> Bus Selector/1, Bus Selector4/1, Bus Selector2/1
  Bus Selector4/1 -> Bus Selector5/1  "<BTMR_flgHtgDrvLogSgns>"
  Bus Selector1/1 -> BTMR_flgHtgDCEna/1  "<BTMR_flgHtgDCEna>"
  BTMR_flgSOCSgns/1 -> Bus Selector6/1
  Bus Selector6/1 -> Logical Operator/2  "<BTMR_flgHtgDrvSOC>"
  Logical Operator/1 -> BTMR_flgHtgDrvEna/1  "BTMR_flgHtgDrvSEna"

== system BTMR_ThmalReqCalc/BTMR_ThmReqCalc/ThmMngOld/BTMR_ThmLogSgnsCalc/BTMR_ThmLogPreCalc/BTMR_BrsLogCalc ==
  BTMR_flgBMSStsSgns : Inport
  BTMR_flgSOCSgns : Inport  Port=2
  BTMR_flgBrsTempSgns : Inport  Port=3
  BTMR_BrsACLogCalc : Subsystem
  BTMR_BrsDCLogCalc : Subsystem
  BTMR_BrsDrvLogCalc : Subsystem
  BTMR_BrsEnaLogCalc : Subsystem
  Bus Creator1 : BusCreator  Inputs=4
  Bus Selector1 : BusSelector  OutputSignals=BTMR_flgBrsEnTempSgns,BTMR_flgBrsIntTempSgns
  BTMR_flgBrsLogSgns : Outport
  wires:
  Bus Selector1/2 -> BTMR_BrsDrvLogCalc/3(BTMR_flgBrsIntSgns), BTMR_BrsACLogCalc/3(BTMR_flgBrsIntSgns), BTMR_BrsDCLogCalc/3(BTMR_flgBrsIntSgns)  "<BTMR_flgBrsIntTempSgns>"
  Bus Selector1/1 -> BTMR_BrsDCLogCalc/2(BTMR_flgBrsEnSgns), BTMR_BrsDrvLogCalc/2(BTMR_flgBrsEnSgns), BTMR_BrsACLogCalc/2(BTMR_flgBrsEnSgns)  "<BTMR_flgBrsEnTempSgns>"
  BTMR_flgBMSStsSgns/1 -> BTMR_BrsDrvLogCalc/1(BTMR_flgBMSStsSgns), BTMR_BrsACLogCalc/1(BTMR_flgBMSStsSgns), BTMR_BrsDCLogCalc/1(BTMR_flgBMSStsSgns)
  BTMR_flgBrsTempSgns/1 -> BTMR_BrsEnaLogCalc/4(BTMR_flgBrsTempSgns), Bus Selector1/1
  BTMR_flgSOCSgns/1 -> BTMR_BrsDrvLogCalc/4(BTMR_flgSOCSgns)
  Bus Creator1/1 -> BTMR_flgBrsLogSgns/1  "BTMR_flgBrsLogSgns"
  BTMR_BrsDCLogCalc/1(BTMR_flgBrsDCLogSgns) -> BTMR_BrsEnaLogCalc/1(BTMR_flgBrsDCLogSgns), Bus Creator1/1
  BTMR_BrsACLogCalc/1(BTMR_flgBrsACLogSgns) -> BTMR_BrsEnaLogCalc/2(BTMR_flgBrsACLogSgns), Bus Creator1/2
  BTMR_BrsDrvLogCalc/1(BTMR_flgBrsDrvLogSgns) -> BTMR_BrsEnaLogCalc/3(BTMR_flgBrsDrvLogSgns), Bus Creator1/3
  BTMR_BrsEnaLogCalc/1(BTMR_flgBrsEnaLogSgns) -> Bus Creator1/4

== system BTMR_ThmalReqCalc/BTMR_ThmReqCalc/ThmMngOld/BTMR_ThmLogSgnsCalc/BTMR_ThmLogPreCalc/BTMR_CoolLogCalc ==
  BTMR_flgHtgLogSgns : Inport
  BTMR_flgThmEnaTempSgns : Inport  Port=2
  BTMR_CoolChrgLogCalc : Subsystem
  BTMR_CoolNormLogCalc : Subsystem
  Bus Creator : BusCreator  Inputs=2
  BTMR_flgCoolLogSgns : Outport
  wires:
  BTMR_flgHtgLogSgns/1 -> BTMR_CoolNormLogCalc/1(BTMR_flgHtgLogSgns), BTMR_CoolChrgLogCalc/1(BTMR_flgHtgLogSgns)
  BTMR_flgThmEnaTempSgns/1 -> BTMR_CoolNormLogCalc/2(BTMR_flgThmEnaTempSgns), BTMR_CoolChrgLogCalc/2(BTMR_flgThmEnaTempSgns)
  BTMR_CoolChrgLogCalc/1(BTMR_flgCoolChrgLogSgns) -> Bus Creator/2
  BTMR_CoolNormLogCalc/1(BTMR_flgCoolNormLogSgns) -> Bus Creator/1
  Bus Creator/1 -> BTMR_flgCoolLogSgns/1  "BTMR_flgCoolLogSgns"

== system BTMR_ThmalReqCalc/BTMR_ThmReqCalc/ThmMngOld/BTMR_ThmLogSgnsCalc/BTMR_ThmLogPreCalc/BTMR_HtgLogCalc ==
  BTMR_flgBrsLogSgns : Inport
  BTMR_flgThmEnaTempSgns : Inport  Port=2
  BTMR_HtgACLogCalc : Subsystem
  BTMR_HtgDCLogCalc : Subsystem
  BTMR_HtgDrvLogCalc : Subsystem
  Bus Creator : BusCreator  Inputs=3
  BTMR_flgHtgLogSgns : Outport
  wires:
  BTMR_HtgDCLogCalc/1(BTMR_flgHtgDCLogSgns) -> Bus Creator/1
  BTMR_flgThmEnaTempSgns/1 -> BTMR_HtgDrvLogCalc/2(BTMR_flgThmEnaTempSgns), BTMR_HtgACLogCalc/2(BTMR_flgThmEnaTempSgns), BTMR_HtgDCLogCalc/2(BTMR_flgThmEnaTempSgns)
  BTMR_HtgDrvLogCalc/1(BTMR_flgHtgDrvLogSgns) -> Bus Creator/3
  Bus Creator/1 -> BTMR_flgHtgLogSgns/1  "BTMR_flgHtgLogSgns"
  BTMR_HtgACLogCalc/1(BTMR_flgHtgACLogSgns) -> Bus Creator/2
  BTMR_flgBrsLogSgns/1 -> BTMR_HtgDrvLogCalc/1(BTMR_flgBrsLogSgns), BTMR_HtgACLogCalc/1(BTMR_flgBrsLogSgns), BTMR_HtgDCLogCalc/1(BTMR_flgBrsLogSgns)

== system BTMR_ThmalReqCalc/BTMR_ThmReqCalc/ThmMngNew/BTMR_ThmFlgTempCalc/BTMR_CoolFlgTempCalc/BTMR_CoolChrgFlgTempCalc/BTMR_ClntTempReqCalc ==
  BTMR_stsClntStg : Inport
  Constant : Constant  Value=BTMR_tChrgClntTempLv1_C
  Constant1 : Constant  Value=BTMR_tChrgClntTempLv2_C
  Constant2 : Constant  Value=BTMR_tChrgClntTempLv3_C
  Constant3 : Constant  Value=0  OutDataTypeStr=single
  Constant6 : Constant  Value=enmThmCoolChrgStg_891.Default  OutDataTypeStr=Enum: enmThmCoolChrgStg_891
  Constant7 : Constant  Value=enmThmCoolChrgStg_891.Stg_Lv1  OutDataTypeStr=Enum: enmThmCoolChrgStg_891
  Constant8 : Constant  Value=enmThmCoolChrgStg_891.Stg_Lv2  OutDataTypeStr=Enum: enmThmCoolChrgStg_891
  Data Type Conversion3 : DataTypeConversion  OutDataTypeStr=uint8
  Data Type Conversion4 : DataTypeConversion  OutDataTypeStr=uint8
  Data Type Conversion5 : DataTypeConversion  OutDataTypeStr=uint8
  Relational Operator : RelationalOperator  Operator=~=  OutDataTypeStr=boolean  RndMeth=Simplest
  Relational Operator1 : RelationalOperator  Operator=~=  OutDataTypeStr=boolean  RndMeth=Simplest
  Relational Operator2 : RelationalOperator  Operator=~=  OutDataTypeStr=boolean  RndMeth=Simplest
  Switch1 : Switch  Criteria=u2 ~= 0
  Switch2 : Switch  Criteria=u2 ~= 0
  Switch3 : Switch  Criteria=u2 ~= 0
  BTMR_tClntTempReq : Outport  InitialOutput=0
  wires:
  BTMR_stsClntStg/1 -> Relational Operator1/1, Relational Operator/1, Relational Operator2/1
  Relational Operator/1 -> Switch1/2
  Switch2/1 -> Switch1/1
  Constant3/1 -> Switch1/3
  Data Type Conversion3/1 -> Relational Operator/2
  Constant6/1 -> Data Type Conversion3/1
  Switch1/1 -> BTMR_tClntTempReq/1
  Switch3/1 -> Switch2/1
  Constant8/1 -> Data Type Conversion5/1
  Relational Operator2/1 -> Switch3/2
  Data Type Conversion5/1 -> Relational Operator2/2
  Relational Operator1/1 -> Switch2/2
  Data Type Conversion4/1 -> Relational Operator1/2
  Constant7/1 -> Data Type Conversion4/1
  Constant/1 -> Switch2/3
  Constant2/1 -> Switch3/1
  Constant1/1 -> Switch3/3

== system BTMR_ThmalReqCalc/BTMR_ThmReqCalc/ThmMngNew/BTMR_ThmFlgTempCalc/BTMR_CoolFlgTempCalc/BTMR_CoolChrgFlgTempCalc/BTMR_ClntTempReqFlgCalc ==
  BTMR_stsClntStg : Inport
  Constant4 : Constant  Value=enmThmCoolFlg.COOL  OutDataTypeStr=Enum: enmThmCoolFlg
  Constant5 : Constant  Value=enmThmCoolFlg.INACTIVE  OutDataTypeStr=Enum: enmThmCoolFlg
  Constant6 : Constant  Value=enmThmCoolNormStg_891.Default  OutDataTypeStr=Enum: enmThmCoolNormStg_891
  Data Type Conversion1 : DataTypeConversion  OutDataTypeStr=uint8
  Data Type Conversion2 : DataTypeConversion  OutDataTypeStr=uint8
  Data Type Conversion3 : DataTypeConversion  OutDataTypeStr=uint8
  Relational Operator : RelationalOperator  Operator=~=  OutDataTypeStr=boolean  RndMeth=Simplest
  Switch : Switch  Criteria=u2 ~= 0
  BTMR_flgClntTempReq : Outport  InitialOutput=0
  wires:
  Data Type Conversion2/1 -> Switch/3
  Data Type Conversion1/1 -> Switch/1
  Constant4/1 -> Data Type Conversion1/1
  Switch/1 -> BTMR_flgClntTempReq/1
  Constant5/1 -> Data Type Conversion2/1
  Data Type Conversion3/1 -> Relational Operator/2
  Constant6/1 -> Data Type Conversion3/1
  BTMR_stsClntStg/1 -> Relational Operator/1
  Relational Operator/1 -> Switch/2

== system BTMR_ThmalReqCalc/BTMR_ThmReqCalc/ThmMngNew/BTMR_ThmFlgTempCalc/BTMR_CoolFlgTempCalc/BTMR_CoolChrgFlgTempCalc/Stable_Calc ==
  source_Uint : Inport
  cntStable : Inport  Port=2
  Chart : Stateflow chart  TreatAsAtomicUnit=on
  Delay1 : Delay  DelayLength=1  InitialCondition=0
  Detect Change : simulink/Logic and Bit Operations/Detect Change  vinit=0  OutDataTypeStr=boolean
  Switch : Switch  Criteria=u2 ~= 0
  stableOut : Outport
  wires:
  source_Uint/1 -> Detect Change/1, Switch/3
  Switch/1 -> stableOut/1, Delay1/1
  Delay1/1 -> Switch/1
  Chart/1(flg_out) -> Switch/2
  cntStable/1 -> Chart/2(cntStable)
  Detect Change/1 -> Chart/1(trigger_in)

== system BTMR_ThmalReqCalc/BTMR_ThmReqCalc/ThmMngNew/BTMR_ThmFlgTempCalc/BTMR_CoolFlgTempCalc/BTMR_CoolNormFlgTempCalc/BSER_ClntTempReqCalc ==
  BTMR_stsClntStg : Inport
  Constant15 : Constant  Value=BTMR_tNormClntTempLv3_C
  Constant3 : Constant  Value=0  OutDataTypeStr=single
  Constant4 : Constant  Value=BTMR_tNormClntTempLv1_C
  Constant5 : Constant  Value=BTMR_tNormClntTempLv2_C
  Constant6 : Constant  Value=enmThmCoolNormStg_891.Default  OutDataTypeStr=Enum: enmThmCoolNormStg_891
  Constant7 : Constant  Value=enmThmCoolNormStg_891.Stg_Lv1  OutDataTypeStr=Enum: enmThmCoolNormStg_891
  Constant8 : Constant  Value=enmThmCoolNormStg_891.Stg_Lv2  OutDataTypeStr=Enum: enmThmCoolNormStg_891
  Data Type Conversion3 : DataTypeConversion  OutDataTypeStr=uint8
  Data Type Conversion4 : DataTypeConversion  OutDataTypeStr=uint8
  Data Type Conversion5 : DataTypeConversion  OutDataTypeStr=uint8
  Relational Operator : RelationalOperator  Operator=~=  OutDataTypeStr=boolean  RndMeth=Simplest
  Relational Operator1 : RelationalOperator  Operator=~=  OutDataTypeStr=boolean  RndMeth=Simplest
  Relational Operator2 : RelationalOperator  Operator=~=  OutDataTypeStr=boolean  RndMeth=Simplest
  Switch1 : Switch  Criteria=u2 ~= 0
  Switch2 : Switch  Criteria=u2 ~= 0
  Switch3 : Switch  Criteria=u2 ~= 0
  BTMR_tClntTempReq : Outport  InitialOutput=0
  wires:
  BTMR_stsClntStg/1 -> Relational Operator1/1, Relational Operator/1, Relational Operator2/1
  Relational Operator/1 -> Switch1/2
  Switch2/1 -> Switch1/1
  Constant3/1 -> Switch1/3
  Data Type Conversion3/1 -> Relational Operator/2
  Constant6/1 -> Data Type Conversion3/1
  Switch1/1 -> BTMR_tClntTempReq/1
  Switch3/1 -> Switch2/1
  Constant8/1 -> Data Type Conversion5/1
  Relational Operator2/1 -> Switch3/2
  Data Type Conversion5/1 -> Relational Operator2/2
  Relational Operator1/1 -> Switch2/2
  Data Type Conversion4/1 -> Relational Operator1/2
  Constant7/1 -> Data Type Conversion4/1
  Constant4/1 -> Switch2/3
  Constant15/1 -> Switch3/1
  Constant5/1 -> Switch3/3

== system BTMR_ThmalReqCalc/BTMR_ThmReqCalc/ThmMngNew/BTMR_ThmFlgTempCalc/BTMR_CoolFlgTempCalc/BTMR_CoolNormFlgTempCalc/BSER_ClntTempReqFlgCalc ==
  BTMR_stsClntStg : Inport
  Constant4 : Constant  Value=enmThmCoolFlg.COOL  OutDataTypeStr=Enum: enmThmCoolFlg
  Constant5 : Constant  Value=enmThmCoolFlg.INACTIVE  OutDataTypeStr=Enum: enmThmCoolFlg
  Constant6 : Constant  Value=enmThmCoolNormStg_891.Default  OutDataTypeStr=Enum: enmThmCoolNormStg_891
  Data Type Conversion1 : DataTypeConversion  OutDataTypeStr=uint8
  Data Type Conversion2 : DataTypeConversion  OutDataTypeStr=uint8
  Data Type Conversion3 : DataTypeConversion  OutDataTypeStr=uint8
  Relational Operator : RelationalOperator  Operator=~=  OutDataTypeStr=boolean  RndMeth=Simplest
  Switch : Switch  Criteria=u2 ~= 0
  BTMR_flgClntTempReq : Outport  InitialOutput=0
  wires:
  Data Type Conversion2/1 -> Switch/3
  Data Type Conversion1/1 -> Switch/1
  Constant4/1 -> Data Type Conversion1/1
  Switch/1 -> BTMR_flgClntTempReq/1
  Constant5/1 -> Data Type Conversion2/1
  Data Type Conversion3/1 -> Relational Operator/2
  Constant6/1 -> Data Type Conversion3/1
  BTMR_stsClntStg/1 -> Relational Operator/1
  Relational Operator/1 -> Switch/2
